(* Logix 5000 AddOnInstructionDefinition export AMCI_NXFE2_Registration_Move_CCW; software revision 20.03 *)

ADD_ON_INSTRUCTION AMCI_NXFE2_Registration_Move_CCW   (* revision 1.0, vendor AMCI, ExecuteEnableInFalse *)
VAR_INPUT
   Type_0_for_standard_1_for_indexed : BOOL;
   Axis_Status_bits : INT; {required}
   _0_normal_1_S_curve_acceleration : BOOL;
   _0_Triangular_1_Trapezoidal_S_Curve : BOOL;
   Stopping_Distance : DINT; {required}
   Programmed_Speed : DINT; {required}
   Acceleration : INT; {required}
   Deceleration : INT; {required}
END_VAR
VAR_OUTPUT
   EN : BOOL; {access Read Only, visible}
   Registration_Move_CCW_Occurring : BOOL; {access Read Only, visible}
   ER : BOOL; {access Read Only, visible}
END_VAR
VAR_IN_OUT
   NXFE2_output_data : _000A:NXFE2_0986AEB4:O:0; {required}
END_VAR
VAR
   command_data_block : INT[10];
        [0]   // Command Bits MSW
        [1]   // Command Bits LSW
        [2]   // Upper Target Position
        [3]   // Lower Target Position
        [4]   // Upper Programmed Speed
        [5]   // Lower Programmed Speed
END_VAR

ROUTINE EnableInFalse   (* ladder *)
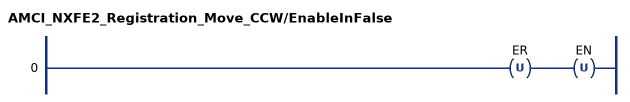
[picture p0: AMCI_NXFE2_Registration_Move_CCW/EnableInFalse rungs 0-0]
   0: OTU(ER)OTU(EN);
END_ROUTINE

ROUTINE Logic   (* ladder *)
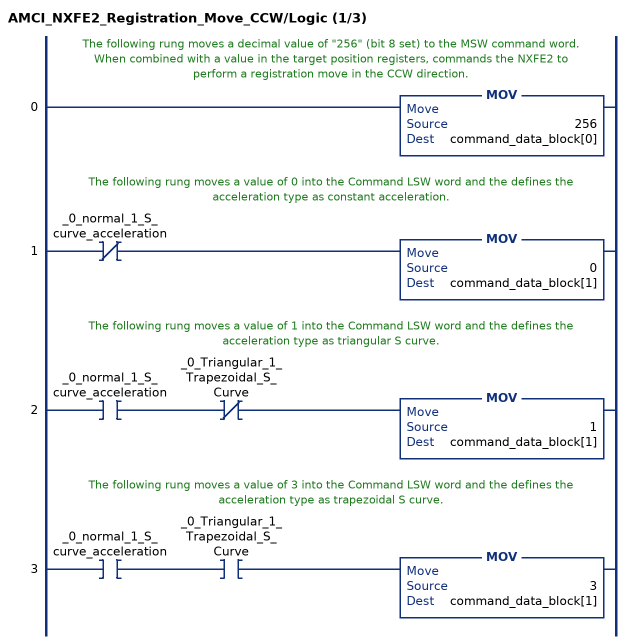
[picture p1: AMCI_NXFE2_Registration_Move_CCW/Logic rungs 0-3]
   // The following rung moves a decimal value of "256" (bit 8 set) to the MSW command word.  When combined with a value in the target position registers, commands the NXFE2 to perform a registration move in the CCW direction.
   0: MOV(256,command_data_block[0]);
   // The following rung moves a value of 0 into the Command LSW word and the defines the acceleration type as constant acceleration.
   1: XIO(_0_normal_1_S_curve_acceleration)MOV(0,command_data_block[1]);
   // The following rung moves a value of 1 into the Command LSW word and the defines the acceleration type as triangular S curve.
   2: XIC(_0_normal_1_S_curve_acceleration)XIO(_0_Triangular_1_Trapezoidal_S_Curve)MOV(1,command_data_block[1]);
   // The following rung moves a value of 3 into the Command LSW word and the defines the acceleration type as trapezoidal S curve.
   3: XIC(_0_normal_1_S_curve_acceleration)XIC(_0_Triangular_1_Trapezoidal_S_Curve)MOV(3,command_data_block[1]);
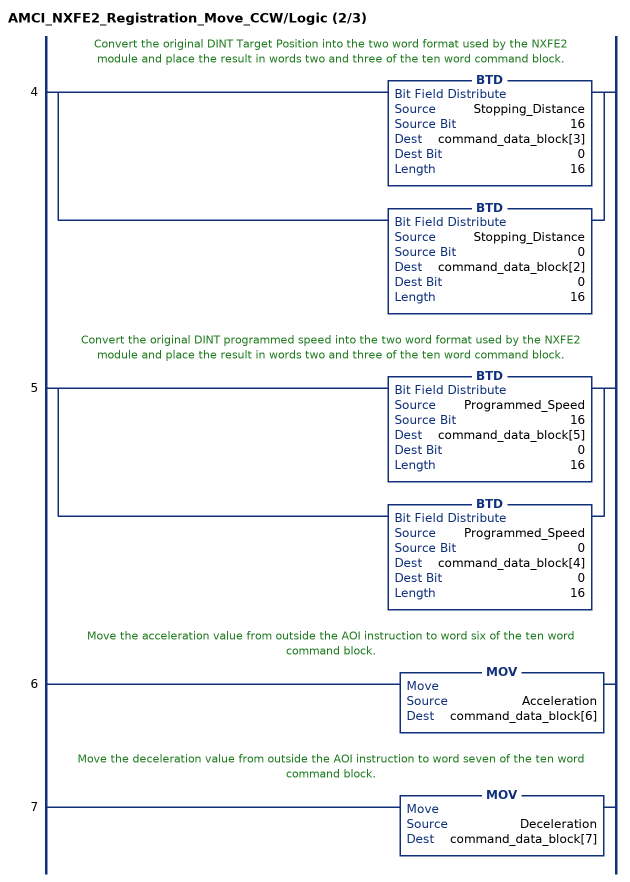
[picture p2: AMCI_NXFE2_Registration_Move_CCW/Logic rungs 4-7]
   // Convert the original DINT Target Position into the two word format used by the NXFE2 module and place the result in words two and three of the ten word command block.
   4: [BTD(Stopping_Distance,16,command_data_block[3],0,16) ,BTD(Stopping_Distance,0,command_data_block[2],0,16) ];
   // Convert the original DINT programmed speed into the two word format used by the NXFE2 module and place the result in words two and three of the ten word command block.
   5: [BTD(Programmed_Speed,16,command_data_block[5],0,16) ,BTD(Programmed_Speed,0,command_data_block[4],0,16) ];
   // Move the acceleration value from outside the AOI instruction to word six of the ten word command block.
   6: MOV(Acceleration,command_data_block[6]);
   // Move the deceleration value from outside the AOI instruction to word seven of the ten word command block.
   7: MOV(Deceleration,command_data_block[7]);
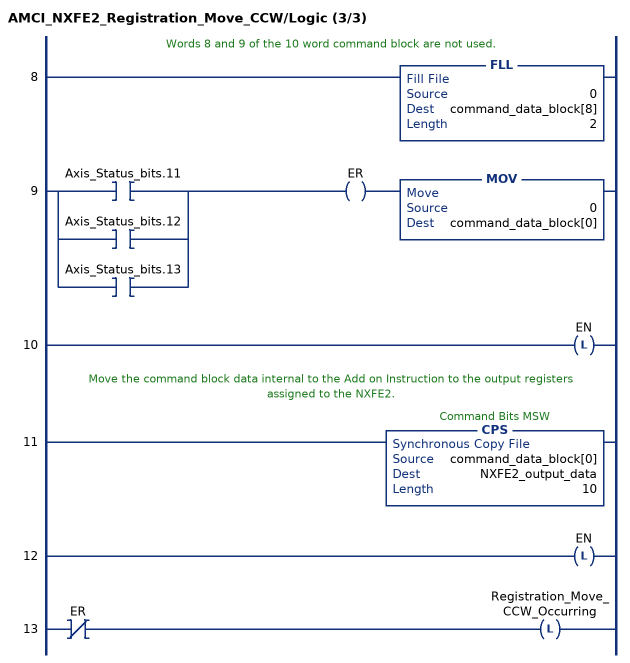
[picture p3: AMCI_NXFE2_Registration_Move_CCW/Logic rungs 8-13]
   // Words 8 and 9 of the 10 word command block are not used.
   8: FLL(0,command_data_block[8],2);
   9: [XIC(Axis_Status_bits.11) ,XIC(Axis_Status_bits.12) ,XIC(Axis_Status_bits.13) ]OTE(ER)MOV(0,command_data_block[0]);
   10: OTL(EN);
   // Move the command block data internal to the Add on Instruction to the output registers assigned to the NXFE2.
   11: CPS(command_data_block[0],NXFE2_output_data,10);
   12: OTL(EN);
   13: XIO(ER)OTL(Registration_Move_CCW_Occurring);
END_ROUTINE
END_ADD_ON_INSTRUCTION
